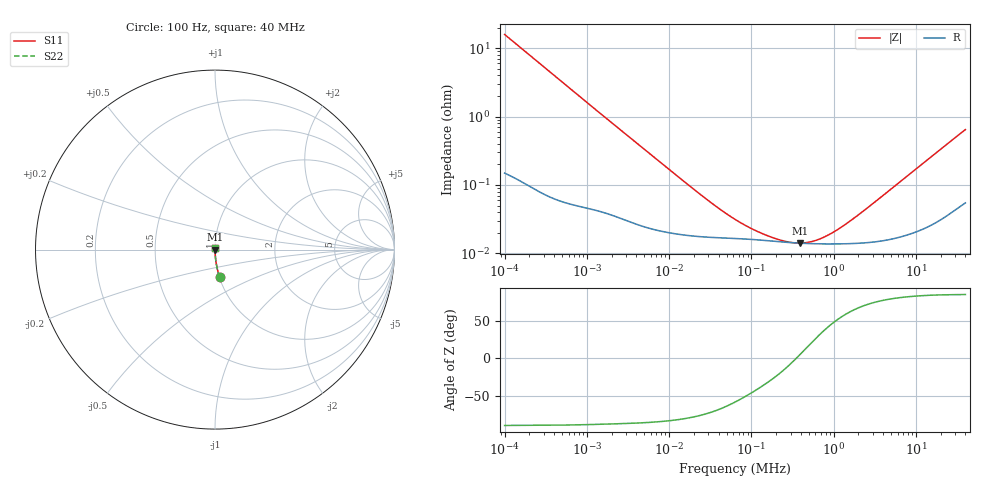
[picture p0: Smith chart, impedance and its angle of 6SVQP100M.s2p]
!  *** S-Parameter ***
!  Copyright (C) Panasonic Industry
!  Conductive Polymer Aluminum Solid Capacitors (OS-CON)
!  Parts No. 6SVQP100M
! Touchstone file from project
# GHZ S RI R 50.000000
! Modal data exported
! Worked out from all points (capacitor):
!   450 points, 100 Hz to 40 MHz, reference 50 ohm
!   read as one part in series: C = 100 uF near 105.9 Hz
!   lowest |Z| = 14.1 mohm at 386.8 kHz (marker M1)
!   series resonance near 350.8 kHz, so ESL is about 2.1 nH
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1e-07  0.0258 -0.154  0.9742 0.154  0.9742 0.154  0.0258 -0.154
1.059254e-07  0.0232 -0.1459  0.9768 0.1459  0.9768 0.1459  0.0232 -0.1459
1.584893e-07  0.011 -0.099  0.989 0.099  0.989 0.099  0.011 -0.099
2.511886e-07  0.00481 -0.063  0.9952 0.063  0.9952 0.063  0.00481 -0.063
4.340103e-07  0.00195 -0.0367  0.998 0.0367  0.998 0.0367  0.00195 -0.0367
8.659643e-07  0.000819 -0.0185  0.9992 0.0185  0.9992 0.0185  0.000819 -0.0185
7.498942e-06  0.000219 -0.00222  0.9998 0.00222  0.9998 0.00222  0.000219 -0.00222
2.985383e-05  0.000172 -0.000567  0.9998 0.000567  0.9998 0.000567  0.000172 -0.000567
4.466836e-05  0.000168 -0.000379  0.9998 0.000379  0.9998 0.000379  0.000168 -0.000379
6.493816e-05  0.000165 -0.00026  0.9998 0.00026  0.9998 0.00026  0.000165 -0.00026
0.0001059254  0.000159 -0.000156  0.9998 0.000156  0.9998 0.000156  0.000159 -0.000156
0.0001727826  0.000152 -8.4e-05  0.9998 8.4e-05  0.9998 8.4e-05  0.000152 -8.4e-05
0.0002660725  0.000145 -3.21e-05  0.9999 3.21e-05  0.9999 3.21e-05  0.000145 -3.21e-05
0.0003868121  0.000141 1.16e-05  0.9999 -1.16e-05  0.9999 -1.16e-05  0.000141 1.16e-05
0.000459727  0.000139 3.26e-05  0.9999 -3.26e-05  0.9999 -3.26e-05  0.000139 3.26e-05
0.0005463865  0.000138 5.49e-05  0.9999 -5.49e-05  0.9999 -5.49e-05  0.000138 5.49e-05
0.0006493816  0.000138 7.91e-05  0.9999 -7.91e-05  0.9999 -7.91e-05  0.000138 7.91e-05
0.0007943282  0.000137 0.00011  0.9999 -0.00011  0.9999 -0.00011  0.000137 0.00011
0.001223207  0.000138 0.000195  0.9999 -0.000195  0.9999 -0.000195  0.000138 0.000195
0.002053525  0.000141 0.000346  0.9999 -0.000346  0.9999 -0.000346  0.000141 0.000346
0.004731513  0.000159 0.000811  0.9998 -0.000811  0.9998 -0.000811  0.000159 0.000811
0.04  0.000588 0.00642  0.9994 -0.00642  0.9994 -0.00642  0.000588 0.00642
